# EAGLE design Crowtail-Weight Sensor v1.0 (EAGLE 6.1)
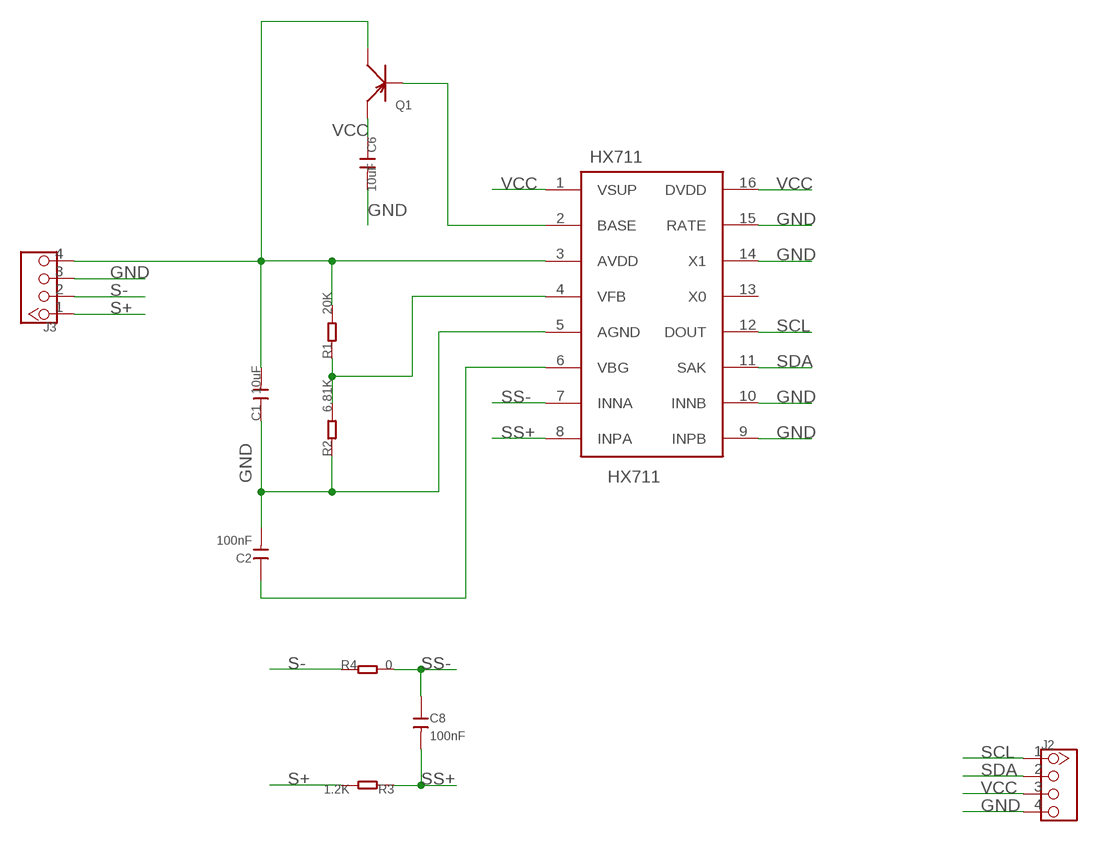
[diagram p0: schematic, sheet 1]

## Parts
C1  10uF  C-0805  [C0805]
C2  100nF  CAP-0603  [C0603]
C6  10uF  C-0805  [C0805]
C8  100nF  CAP-0603  [C0603]
HX711  HX711  [SOP16-L]
J2  TWIG-4P-2.0-2.0  [4P-2.0]
J3  TWIG-4P-2.0-2.0  [4P-2.0]
Q1  TRANSISTOR-PNP-SOT23  [SOT23]
R1  20K  R-0603  [R0603]
R2  6.81K  R-0603  [R0603]
R3  1.2K  R-0603  [R0603]
R4  0  R-0603  [R0603]

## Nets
GND: C1.1 C2.2 C6.2 HX711.5(AGND) HX711.9(INPB) HX711.10(INNB) HX711.14(X1) HX711.15(RATE) J2.4 J3.3 R2.1
N$1: HX711.2(BASE) Q1.1(B)
N$3: C1.2 HX711.3(AVDD) J3.4 Q1.3(C) R1.2
N$4: HX711.4(VFB) R1.1 R2.2
N$5: C2.1 HX711.6(VBG)
S+: J3.1 R3.2
S-: J3.2 R4.1
SCL: HX711.12(DOUT) J2.1
SDA: HX711.11(SAK) J2.2
SS+: C8.2 HX711.8(INPA) R3.1
SS-: C8.1 HX711.7(INNA) R4.2
VCC: C6.1 HX711.1(VSUP) HX711.16(DVDD) J2.3 Q1.2(E)
Unconnected: HX711.13(X0)

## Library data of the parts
C1 C6 = Discrete:C*: Ceramic Capacitors
C2 C8 = Discrete-new:CAP: Ceramic Capacitors
HX711 = IC:HX711
J2 J3 = Connector:TWIG-4P-2.0
Q1 = Discrete:TRANSISTOR-PNP*: PNP audion
R1-R4 = Discrete:R*

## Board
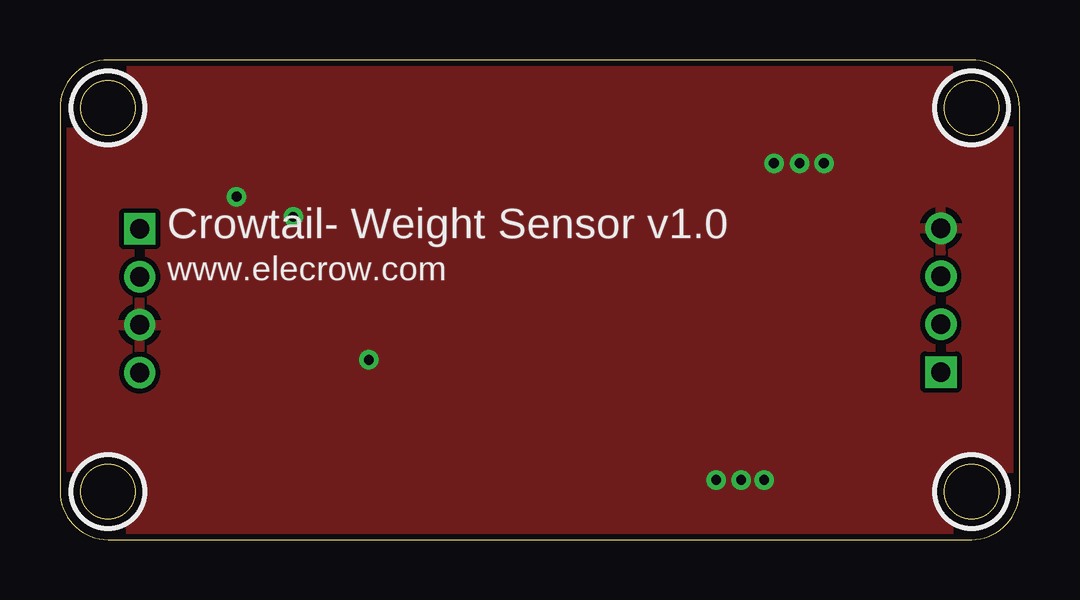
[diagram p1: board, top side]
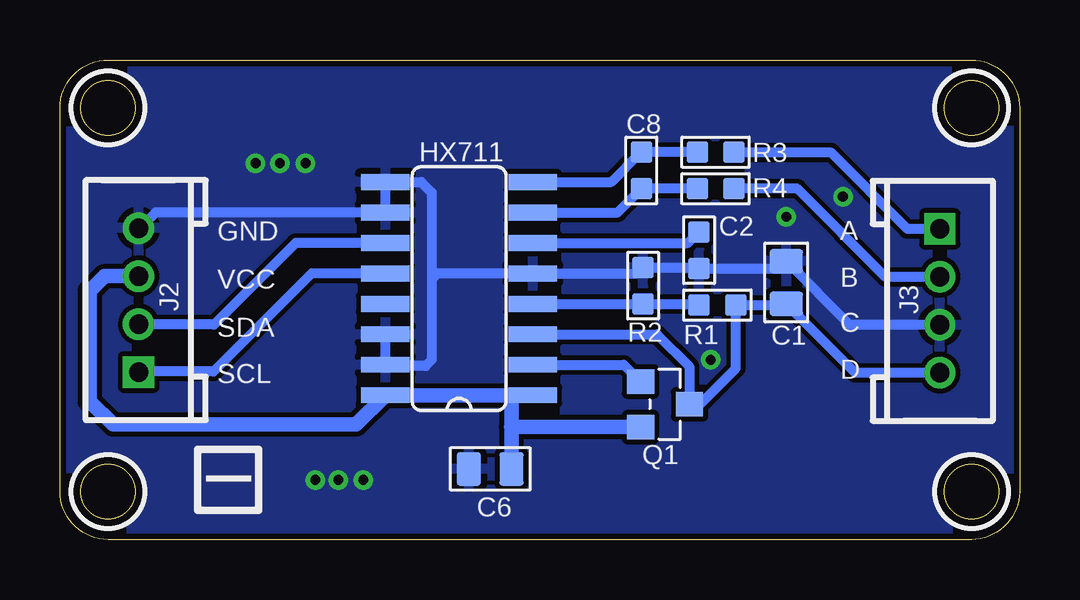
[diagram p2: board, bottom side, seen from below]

Size 40 x 20 mm. Coordinates in mm from the lower left corner, seen from the top.
Outline: 38,20 2,20 arc90 0,18 0,2 arc90 2,0 38,0 arc90 40,2 40,18 arc90 38,20
Outline: circle at 2,18 radius 1.14
Outline: circle at 2,2 radius 1.14
Outline: circle at 38,18 radius 1.14
Outline: circle at 38,2 radius 1.14
Copper layers (1*16): Top 0.035mm / dielectric 1.5mm / Bottom 0.035mm
Design rules: minimum track width 10mil, minimum drill 10mil, track to track 8mil, track to pad 8mil, pad to pad 8mil, via to via 8mil, smd to smd 8mil, copper to edge 10mil, drill to drill 8mil, minimum pad ring 10mil, minimum via ring 8mil, stop-mask expansion 4mil, vias tented up to drill 0mil, thermal gap 10mil
tRestrict: area 0.5,16.5 to 3.5,19.5; area 0.5,0.5 to 3.5,3.5; area 36.5,16.5 to 39.5,19.5; area 36.5,0.5 to 39.5,3.5
bRestrict: area 0.5,16.5 to 3.5,19.5; area 0.5,0.5 to 3.5,3.5; area 36.5,16.5 to 39.5,19.5; area 36.5,0.5 to 39.5,3.5

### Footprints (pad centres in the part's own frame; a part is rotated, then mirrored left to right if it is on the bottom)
C0805 = smd 1.016 x 1.397: 1 -0.889,0; 2 0.889,0
C0603 = smd 0.889 x 0.889: 1 0,0.762; 2 0,-0.762
SOP16-L = smd 0.66 x 2.032: 1 -4.445,-3.073; 2 -3.175,-3.073; 3 -1.905,-3.073; 4 -0.635,-3.073; 5 0.635,-3.073; 6 1.905,-3.073; 7 3.175,-3.073; 8 4.445,-3.073; 9 4.445,3.073; 10 3.175,3.073; 11 1.905,3.073; 12 0.635,3.073; 13 -0.635,3.073; 14 -1.905,3.073; 15 -3.175,3.073; 16 -4.445,3.073
4P-2.0 = drill 0.8 pad 1.27 square: 1 -3,0 | drill 0.8 pad 1.27: 2 -1,0; 3 1,0; 4 3,0
SOT23 = smd 1.016 x 1.143: 1 -0.95,-1.016; 2 0.95,-1.016; 3 0,1.016
R0603 = smd 0.889 x 0.889: 1 -0.762,0; 2 0.762,0

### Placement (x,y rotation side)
C1  9.72,10.72 270 bottom
C2  13.36,12.06 0 bottom
C6  22.07,2.95 180 bottom
C8  15.77,15.39 180 bottom
HX711  23.36,10.46 90 bottom
J2  36.72,9.98 90 bottom
J3  3.32,9.96 270 bottom
Q1  14.78,5.64 270 bottom
R1  12.59,9.78 0 bottom
R2  15.69,10.59 270 bottom
R3  12.67,16.15 0 bottom
R4  12.67,14.63 180 bottom

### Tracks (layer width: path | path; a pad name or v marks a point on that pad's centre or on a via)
GND  (via drill 0.41)
  Bottom 0.406: 24.51,10.85 24.51,14.48 24.94,14.91 HX711.9 HX711.10 36.01,13.64 36.7,12.95 36.7,12.96 J2.4 | 24.51,10.85 24.51,7.49 24.76,7.24 26.39,7.24 HX711.15 HX711.14 | 24.51,10.85 24.25,11.1 HX711.5 15.95,11.1 R2.1 13.41,11.35 C2.2 10.03,11.3 C1.1 | J3.3 7.07,8.96 C1.1 | C1.1 9.72,11.58
  other vias: 9.72,13.46 7.36,14.3 12.87,7.49 30.83,15.7 29.76,15.7 31.85,15.7 29.36,2.49 28.39,2.49 27.35,2.49
  pour Bottom: -0.76,2.79 -0.76,18.29 arc-90 1.52,20.57 38.35,20.57 arc-90 40.64,18.29 40.64,2.03 arc-90 37.85,-0.76 2.79,-0.76 arc-90
  pour Top: -0.76,2.79 -0.76,18.57 arc-90 1.24,20.57 38.86,20.57 arc-90 40.64,18.8 40.64,2.03 arc-90 37.85,-0.76 2.79,-0.76 arc-90
N$1
  Bottom 0.406: HX711.2 16.5,7.29 Q1.1
N$3
  Bottom 0.406: HX711.3 15.11,8.56 13.76,7.21 Q1.3 13.33,5.64 11.83,7.14 R1.2 9.77,9.78 C1.2 6.85,6.96 J3.4
N$4
  Bottom 0.406: HX711.4 R2.2 13.41,9.83 R1.1
N$5
  Bottom 0.406: HX711.6 13.81,12.37 C2.1
S+
  Bottom 0.406: J3.1 4.67,12.96 7.84,16.13 11.88,16.13 R3.2
S-
  Bottom 0.406: J3.2 5.59,10.96 9.27,14.63 R4.1
SCL
  Bottom 0.406: HX711.12 29.51,11.1 33.6,7.01 36.7,7.01 J2.1
SDA
  Bottom 0.406: HX711.11 30.17,12.37 33.57,8.97 36.71,8.97 J2.2
SS+
  Bottom 0.406: R3.1 C8.2 15.79,16.15 15.79,16.13 17.01,14.91 HX711.8
SS-
  Bottom 0.406: R4.2 C8.1 16.76,13.64 HX711.7
VCC
  Bottom 0.406: 21.18,5.87 21.33,6.02 | 21.19,4.69 21.23,4.72 21.23,5.74 21.18,5.79
  Bottom 0.61: HX711.1 21.33,6.02 HX711.16 27.66,4.8 37.79,4.8 38.76,5.77 38.76,10.36 38.14,10.98 J2.3 | C6.1 21.18,5.79 21.18,5.87 | Q1.2 21.19,4.69

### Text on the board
tPlace: Crowtail- Weight Sensor v1.0 | www.elecrow.com
bPlace: A | GND | B | VCC | C | SDA | D | SCL | I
